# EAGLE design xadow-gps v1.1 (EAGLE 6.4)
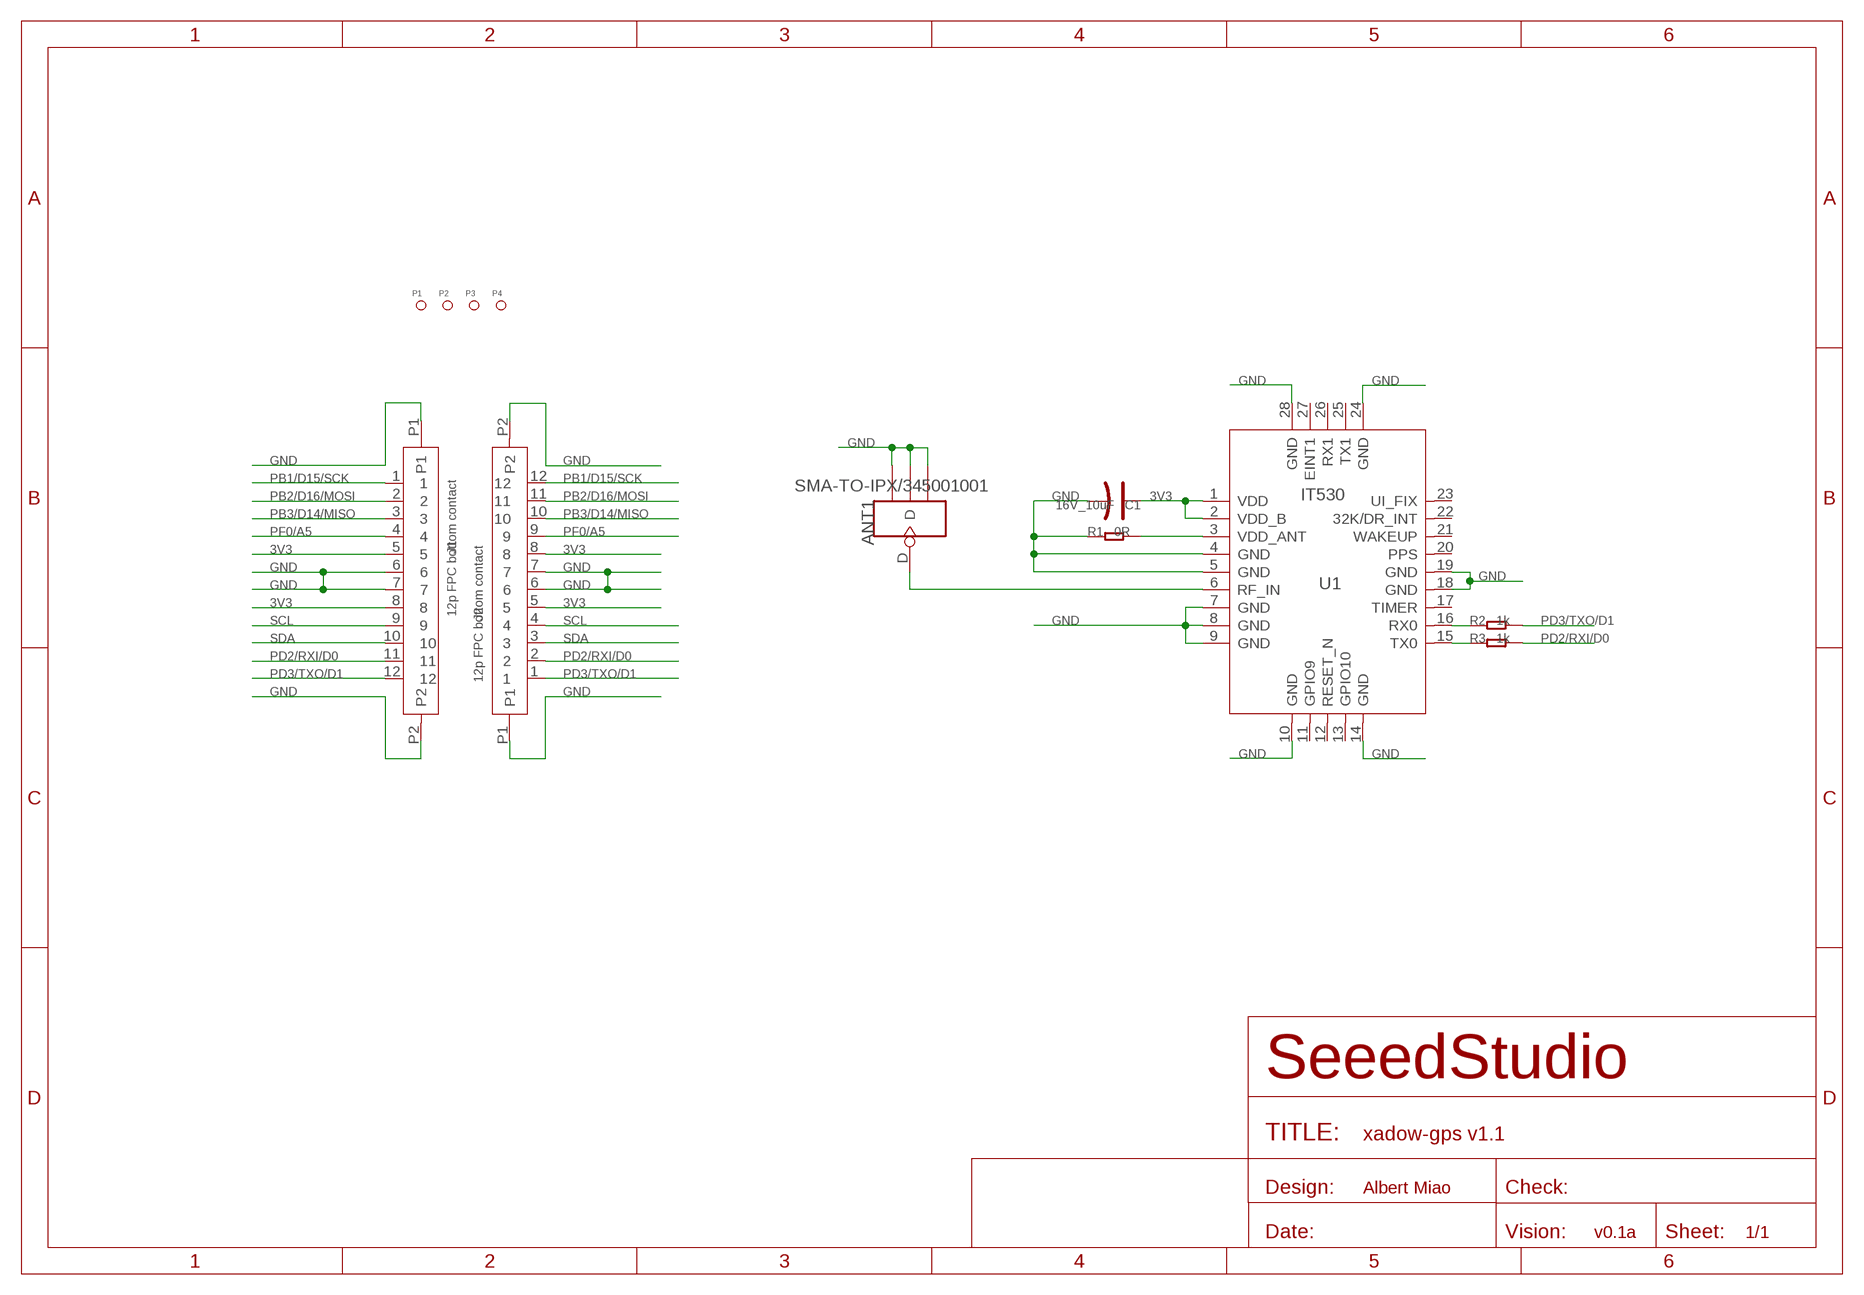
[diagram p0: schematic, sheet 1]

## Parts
ANT1  SMA-TO-IPX/345001001  ANTENNA-U-FL  [4P-U-FL]
C1  16V_10uF  CAP-AVX-A  [AVX-A]
J1  12p FPC bottom contact  FPC052002-12LT  [12P-0.5]
J2  12p FPC bottom contact  FPC052002-12LT  [12P-0.5]
P1  PAD-MARK  [ROUND-MARK-1.0]
P2  PAD-MARK  [ROUND-MARK-1.0]
P3  PAD-MARK  [ROUND-MARK-1.0]
P4  PAD-MARK  [ROUND-MARK-1.0]
R1  0R  R-0603  [R0603]
R2  1k  R-0603  [R0603]
R3  1k  R-0603  [R0603]
U1  IT530  [QFP28]

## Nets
3V3: C1.+ J1.5 J1.8 J2.5 J2.8 U1.1(VDD) U1.2(VDD_B)
GND: ANT1.GND1 ANT1.GND2 ANT1.GND3 C1.- J1.6 J1.7 J1.P1 J1.P2 J2.6 J2.7 J2.P1 J2.P2 R1.1 U1.4(GND) U1.5(GND) U1.7(GND) U1.8(GND) U1.9(GND) U1.10(GND) U1.14(GND) U1.18(GND) U1.19(GND) U1.24(GND) U1.28(GND)
N$1: ANT1.D U1.6(RF_IN)
N$2: R2.1 U1.16(RX0)
N$3: R3.1 U1.15(TX0)
PB1/D15/SCK: J1.1 J2.12
PB2/D16/MOSI: J1.2 J2.11
PB3/D14/MISO: J1.3 J2.10
PD2/RXI/D0: J1.11 J2.2 R3.2
PD3/TXO/D1: J1.12 J2.1 R2.2
PF0/A5: J1.4 J2.9
SCL: J1.9 J2.4
SDA: J1.10 J2.3
VDD_ANT: R1.2 U1.3(VDD_ANT)
Unconnected: U1.11(GPIO9) U1.12(RESET_N) U1.13(GPIO10) U1.17(TIMER) U1.20(PPS) U1.21(WAKEUP) U1.22(32K/DR_INT) U1.23(UI_FIX) U1.25(TX1) U1.26(RX1) U1.27(EINT1)

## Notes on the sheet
- Albert Miao
- v0.1a

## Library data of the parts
ANT1 = Connector:ANTENNA-U-FL
C1 = Discrete:CAP*: Electrolytic Capacitors,Tantalum Capacitors and Super Capacitors
J1 J2 = template:FPC052002-12LT
P1-P4 = Discrete:PAD-MARK; PARTNO: DNP
R1-R3 = Discrete:R*
U1 = For_Test_Albert:IT530: Fastrax miniature GPS module

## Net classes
0 default: width 0.152 mm, drill 0.305 mm, clearance 0.152 mm
1 GND: width 0.152 mm, drill 0.305 mm, clearance 0.152 mm to class 0, clearance 0.152 mm
3 usbvcc: width 0.203 mm, drill 0.305 mm, clearance 0.203 mm

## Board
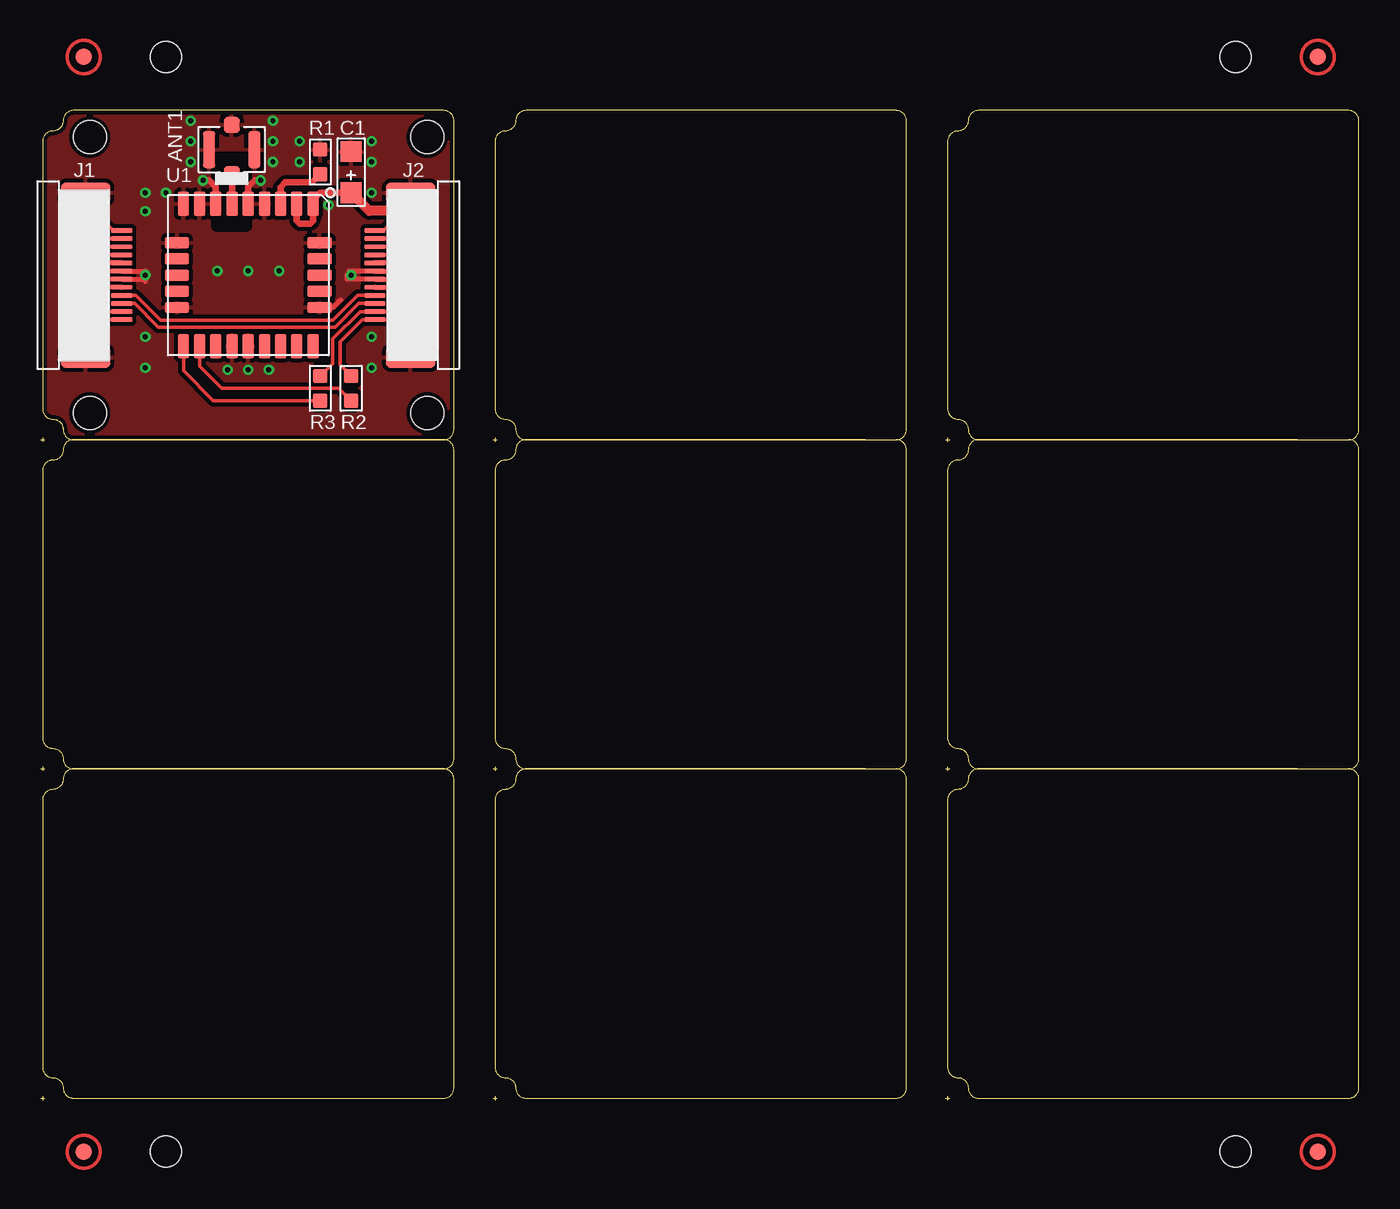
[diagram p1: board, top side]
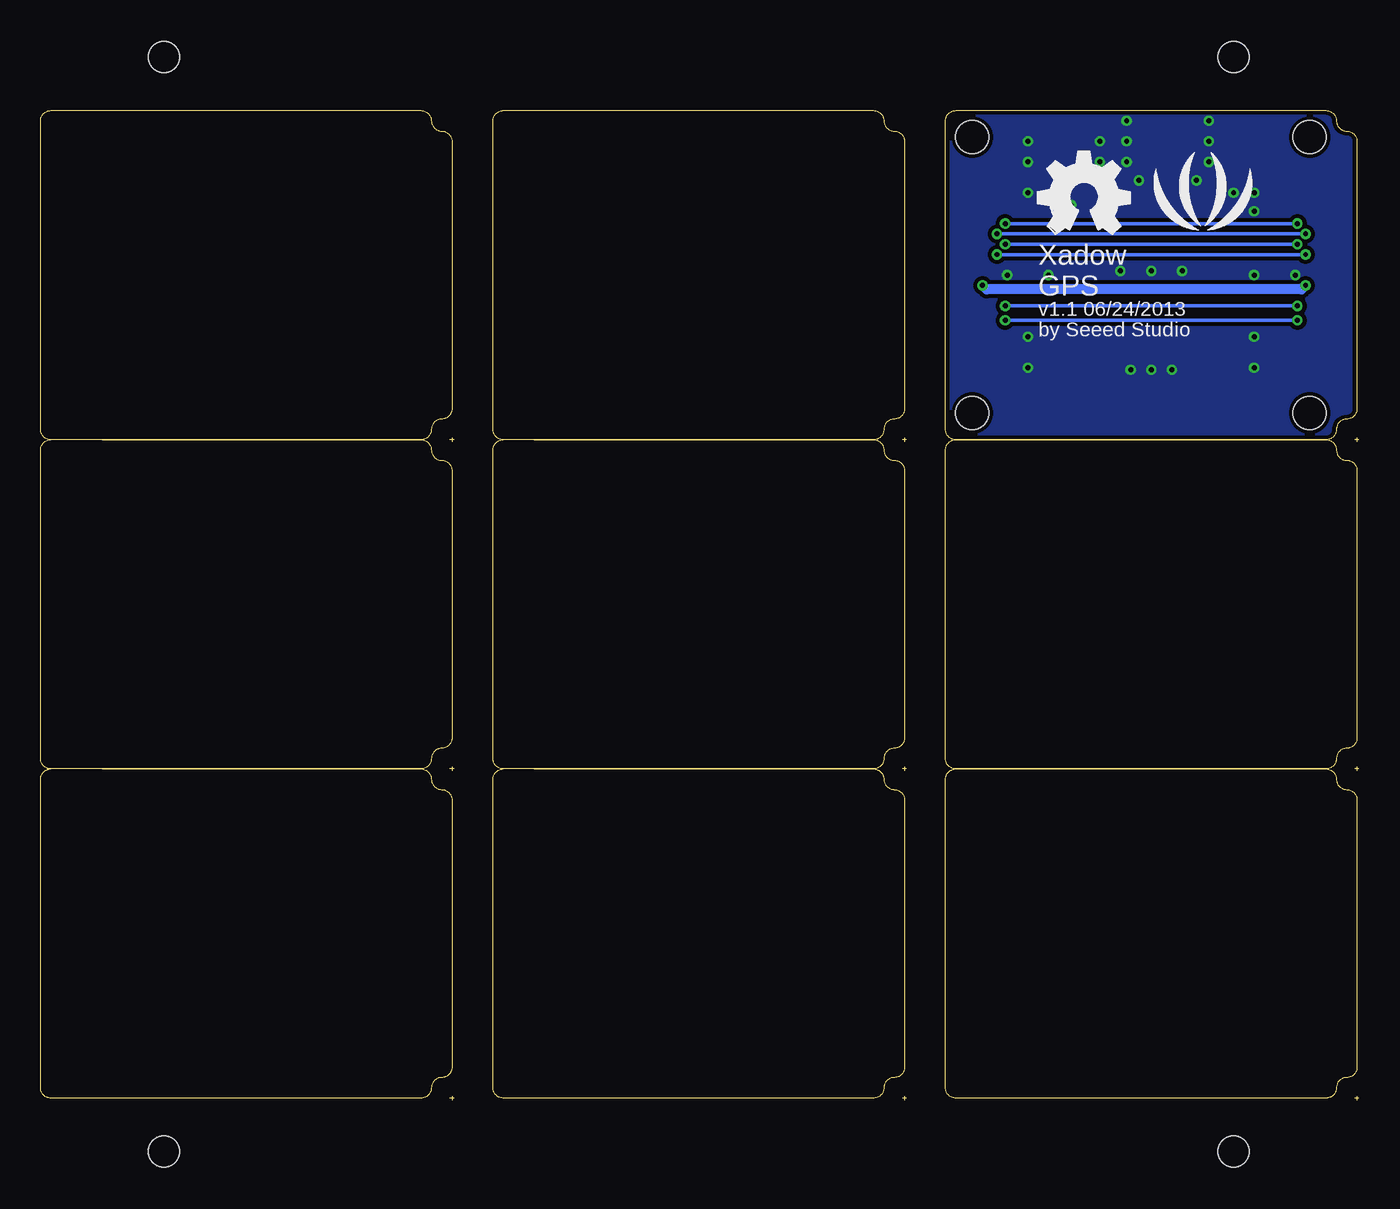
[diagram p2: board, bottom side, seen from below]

Size 81.41 x 61.09 mm. Coordinates in mm from the lower left corner, seen from the top.
Outline: 141 segments
Copper layers (1*16): Top 0.035mm / dielectric 1.5mm / Bottom 0.035mm
Design rules "SeeedStudio_rule_no_angle_090911 *": minimum track width 6mil, minimum drill 12mil, track to track 6mil, track to pad 6mil, pad to pad 6mil, via to via 6mil, smd to smd 0mil, copper to edge 10mil, drill to drill 10mil, minimum pad ring 10mil, minimum via ring 6mil, stop-mask expansion 2mil, vias tented up to drill 100mil, thermal gap 10mil
Holes 2.03 mm at 3.05,42.42 3.05,59.44 23.88,59.44 23.88,42.42
Holes 1.91 mm at 73.79,64.39 7.75,64.39 7.75,-3.17 73.79,-3.17
tRestrict: area 20.1,50.5 to 21.2,51.3; area 4.4,50.5 to 5.6,51.3; area 10.9,47.1 to 11.3,47.5; area 12.2,46.2 to 12.4,46.9; area 9.1,55 to 9.4,55.6; 4 lines

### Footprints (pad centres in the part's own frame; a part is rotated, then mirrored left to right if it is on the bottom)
4P-U-FL = smd 1.016 x 1.016: D -1.524,0; GND3 1.524,0 | smd 2.286 x 0.762: GND1 0,1.397; GND2 0,-1.397
AVX-A = smd 1.27 x 1.27: + -1.27,0; - 1.27,0
12P-0.5 = smd 0.3 x 1.3: 1 -2.75,2.35; 2 -2.25,2.35; 3 -1.75,2.35; 4 -1.25,2.35; 5 -0.75,2.35; 6 -0.25,2.35; 7 0.25,2.35; 8 0.75,2.35; 9 1.25,2.35; 10 1.75,2.35; 11 2.25,2.35; 12 2.75,2.35 | smd 1.27 x 3.048: P1 -5.08,0.127; P2 5.08,0.127
ROUND-MARK-1.0 = smd 1.016 x 1.016: P$1 0,0
R0603 = smd 0.889 x 0.889: 1 -0.762,0; 2 0.762,0
QFP28 = smd 0.7 x 1.5: 1 -4,-4.4; 2 -3,-4.4; 3 -2,-4.4; 4 -1,-4.4; 5 0,-4.4; 6 1,-4.4; 7 2,-4.4; 8 3,-4.4; 9 4,-4.4; 15 4,4.4; 16 3,4.4; 17 2,4.4; 18 1,4.4; 19 0,4.4; 20 -1,4.4; 21 -2,4.4; 22 -3,4.4; 23 -4,4.4 | smd 1.5 x 0.7: 10 4.4,-2; 11 4.4,-1; 12 4.4,0; 13 4.4,1; 14 4.4,2; 24 -4.4,2; 25 -4.4,1; 26 -4.4,0; 27 -4.4,-1; 28 -4.4,-2

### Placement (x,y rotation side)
ANT1  11.81,58.67 90 top
C1  19.18,57.28 90 top
J1  2.67,50.93 270 top
J2  22.99,50.93 90 top
P1  not placed on the board
P2  not placed on the board
P3  not placed on the board
P4  not placed on the board
R1  17.27,57.91 270 top
R2  19.18,43.94 90 top
R3  17.27,43.94 90 top
U1  12.83,50.93 180 top
U$2  [LOGO_SILK]  9.65,55.37 0 bottom
U$3  [OSHW_FILLX200_NOTEXT]  19.81,53.47 0 bottom

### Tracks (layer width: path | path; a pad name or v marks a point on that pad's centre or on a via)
3V3  (via drill 0.3 pad 0.64)
  Top 0.305: 5,50.16 J1.8 3.42,50.18 v3.3,50.29 3.3,51.31 3.67,51.68 J1.5 | J2.8 21.98,51.68 22.23,51.44 22.86,51.44 | 23.13,50.18 v23.24,50.29 22.99,50.04 21.72,50.04 21.58,50.18 J2.5 | 22.86,51.44 23.24,51.44 | 22.86,51.44 23.11,51.69 | 22.86,51.44 23.11,51.18
  Top 0.406: U1.2 15.83,54.28 16,54.1 16.65,54.1 16.83,54.28 U1.1 16.83,55.56 17.27,56.01 C1.+
  Top 0.61: v23.24,50.29 23.24,51.44 23.24,54.36 22.71,54.89 20.3,54.89 C1.+
  Bottom 0.61: v3.3,50.29 3.56,50.04 22.99,50.04 v23.24,50.29
GND  (via drill 0.3 pad 0.64)
  Top 0.305: 6.48,51.18 J1.6 4.19,51.18 v3.94,50.93 4.19,50.68 J1.7 6.48,50.68 6.48,50.55 | 19.05,51.18 J2.7 21.47,51.18 v21.72,50.93 21.47,50.68 J2.6 18.92,50.68 18.92,50.93 | U1.24 18.07,48.93 18.54,49.4
  Top 0.406: U1.7 10.83,56.36 10.41,56.77 v10.03,56.77 | U1.5 12.83,56.39 13.21,56.77 v13.59,56.77
  other vias: 14.35,57.91 14.35,59.18 9.27,57.91 9.27,59.18 10.92,51.18 12.83,51.18 14.73,51.18 11.56,45.09 12.83,45.09 6.48,50.93 19.18,50.93 16,59.18 16,57.91 20.45,57.91 20.45,59.18 6.48,56.01 7.75,56.01 14.1,45.09 6.48,54.86 6.48,45.21 6.48,47.12 20.45,47.12 20.45,45.21 9.27,60.45 14.35,60.45 17.78,55.24 20.45,56.01
  pour Top (isolate 0.254): 0.13,40.77 25.53,40.77 25.53,61.09 0.13,61.09
  pour Bottom (isolate 0.254): 0.13,40.77 25.53,40.77 25.53,61.09 0.13,61.09
N$1
  Top 0.406: U1.6 11.83,57.13 ANT1.D
N$2
  Top 0.203: R2.1 18.41,43.94 11.18,43.94 9.83,45.29 U1.16
N$3
  Top 0.203: U1.15 8.83,45.02 10.67,43.18 R3.1
PB1/D15/SCK  (via drill 0.3 pad 0.64)
  Top 0.203: v3.81,54.1 4.06,54.1 4.45,53.72 4.97,53.72 J1.1 | v21.84,54.1 21.59,54.1 21.21,53.72 20.68,53.72 J2.12
  Bottom 0.203: v3.81,54.1 v21.84,54.1
PB2/D16/MOSI  (via drill 0.3 pad 0.64)
  Top 0.203: 4.99,53.15 J1.2 4.29,53.18 4,53.47 v3.3,53.47 | v22.35,53.47 21.59,53.47 21.3,53.18 J2.11
  Bottom 0.203: v22.35,53.47 v3.3,53.47
PB3/D14/MISO  (via drill 0.3 pad 0.64)
  Top 0.203: J1.3 4.28,52.68 4.13,52.83 v3.81,52.83 | v21.84,52.83 21.46,52.83 21.31,52.68 J2.10
  Bottom 0.203: v3.81,52.83 v21.84,52.83
PD2/RXI/D0  (via drill 0.3 pad 0.64)
  Top 0.203: R3.2 18.03,45.47 18.03,46.99 19.72,48.68 J2.2 21.5,48.68 v21.84,49.02 | J1.11 4.15,48.68 v3.81,49.02
  Bottom 0.203: v3.81,49.02 v21.84,49.02
PD3/TXO/D1  (via drill 0.3 pad 0.64)
  Top 0.203: J1.12 3.85,48.18 v3.81,48.13 | v21.84,48.13 21.8,48.18 J2.1 19.86,48.18 18.5,46.82 18.5,45.38 R2.2
  Bottom 0.203: v3.81,48.13 v21.84,48.13
PF0/A5  (via drill 0.3 pad 0.64)
  Top 0.203: v3.3,52.2 5,52.2 J1.4 | v22.35,52.2 20.66,52.2 J2.9
  Bottom 0.203: v22.35,52.2 v3.3,52.2
SCL
  Top 0.203: J2.4 19.58,49.68 18.04,48.13 7.43,48.13 5.89,49.68 J1.9
SDA
  Top 0.203: J2.3 19.65,49.18 18.19,47.72 7.28,47.72 5.81,49.18 J1.10
VDD_ANT
  Top 0.406: U1.3 14.83,56.36 15.11,56.64 16.76,56.64 R1.2

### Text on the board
bPlace: Xadow | GPS | v1.1 06/24/2013 | by Seeed Studio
